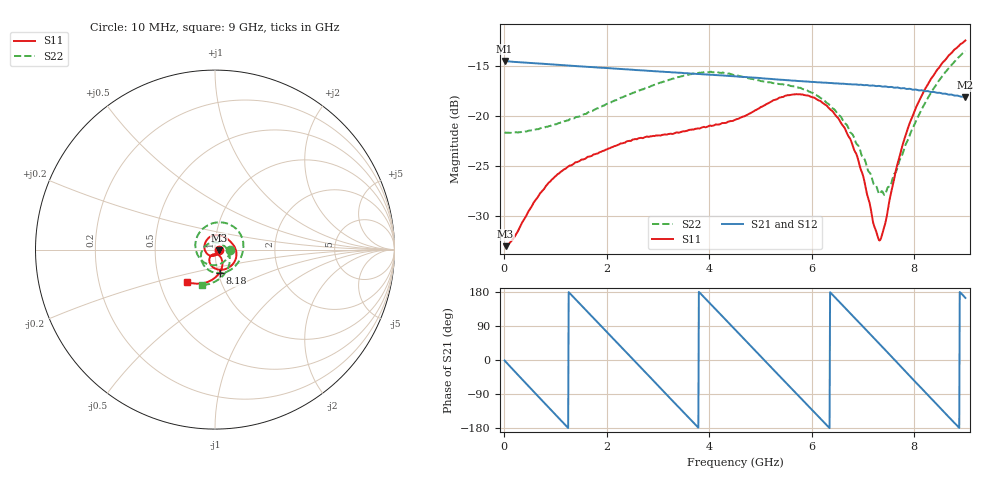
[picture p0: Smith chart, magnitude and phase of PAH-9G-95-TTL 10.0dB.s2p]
! MTS Systemtechnik GmbH
! S-Parameters
! Model: PAH-9G/95-TTL
! Attenuation Step: 10.0dB
#  HZ  S  DB  R  50.00
! Rohde & Schwarz Vector Network Analyzer
! Rohde-Schwarz,ZNB20-2Port,1334333062101652,3.45
! Created: UTC 1/26/2024, 7:19:21 AM
! freq[Hz]  db:S11  ang:S11  db:S21  ang:S21  db:S12  ang:S12  db:S22  ang:S22
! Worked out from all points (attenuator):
!   900 points, 10 MHz to 9 GHz, reference 50 ohm
!   highest |S21| = -14.50 dB at 10 MHz (marker M1); lowest = -18.1 dB at 9 GHz (marker M2)
!   lowest |S11| = -33.0 dB at 30 MHz (marker M3), VSWR 1.05, Z = 52.3 - j0.387 ohm
!   |S11| at or under -10 dB: start of sweep to end of sweep
!   |S22| runs from -27.9 to -13.5 dB; largest |S21 - S12| = 0.0056
!   S11 on the Smith chart (normalised r, x): 10 MHz: 1.05, -0.01; 8.18 GHz: 1.02, -0.27; 9 GHz: 0.69, -0.26
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1e7  -32.92 -8.4  -14.50 -1.4  -14.50 -1.4  -21.62 -3.0
3e7  -33.02 -9.6  -14.52 -4.5  -14.53 -4.5  -21.68 -4.5
3.9e8  -30.36 -78.2  -14.66 -56.6  -14.67 -56.5  -21.57 -47.8
6.9e8  -27.83 -119.3  -14.76 -99.6  -14.77 -99.5  -21.28 -82.7
1.12e9  -25.54 -162.7  -14.91 -160.9  -14.93 -160.8  -20.64 -126.9
1.51e9  -24.37 168.6  -15.06 143.6  -15.06 143.8  -19.92 -161.3
1.93e9  -23.50 143.2  -15.19 84.1  -15.19 84.3  -18.98 167.3
2.39e9  -22.54 118.1  -15.34 18.8  -15.35 19.5  -17.94 136.3
3.01e9  -21.95 88.8  -15.55 -68.5  -15.56 -68.5  -16.75 98.3
3.35e9  -21.68 74.3  -15.66 -116.8  -15.66 -116.2  -16.20 78.3
3.77e9  -21.25 57.6  -15.80 -175.8  -15.80 -175.4  -15.72 52.8
4.51e9  -20.39 29.5  -16.04 79.8  -16.05 80.1  -15.90 8.0
5.16e9  -18.72 -0.8  -16.28 -12.2  -16.30 -11.2  -16.63 -28.9
5.6e9  -17.88 -29.0  -16.46 -74.2  -16.47 -73.2  -17.01 -56.3
6.01e9  -18.13 -59.6  -16.59 -132.0  -16.61 -130.8  -17.67 -87.1
6.37e9  -19.38 -87.4  -16.71 177.5  -16.73 178.4  -19.00 -118.7
6.75e9  -22.27 -113.8  -16.82 123.8  -16.85 124.8  -21.60 -158.4
7.31e9  -32.37 -91.9  -17.00 44.5  -17.04 45.3  -27.76 107.4
7.51e9  -28.68 -57.6  -17.12 16.0  -17.12 17.1  -27.09 56.9
7.8e9  -22.47 -57.7  -17.22 -25.6  -17.29 -24.2  -23.39 0.6
8.18e9  -17.64 -78.9  -17.48 -80.1  -17.53 -78.0  -19.01 -44.2
9e9  -12.45 -131.0  -18.13 163.8  -18.18 165.7  -13.50 -110.4
